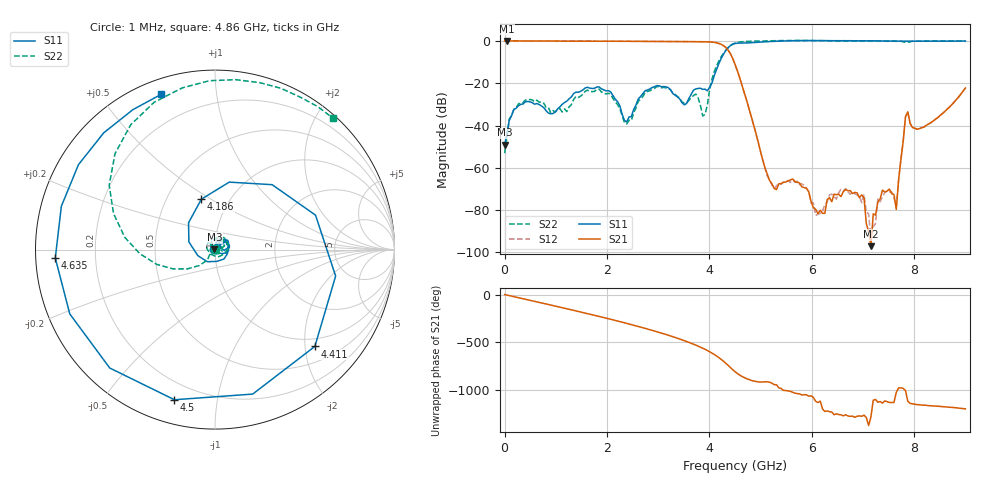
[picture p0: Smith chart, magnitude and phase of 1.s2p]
!Prosund Technologies,SP809B,SP82221046,V.03.04.C
!Date: Sunday, January 19, 2025 15:10:32
!Correction: S11(C  2-Port  )
!S21(C  2-Port  )
!S12(C  2-Port  )
!S22(C  2-Port  )
!S2P File: Measurement: :
# Hz S  dB  R 50
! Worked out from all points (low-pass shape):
!   201 points, 1 MHz to 9 GHz, reference 50 ohm
!   highest |S21| = 0.01 dB at 45.99 MHz (marker M1); lowest = -97.0 dB at 7.155 GHz (marker M2)
!   |S21| within 3 dB of the highest: start of sweep to 4.314 GHz
!   lowest |S11| = -49.0 dB at 1 MHz (marker M3), VSWR 1.01, Z = 49.7 + j0.187 ohm
!   |S11| at or under -10 dB: start of sweep to 4.199 GHz
!   |S22| runs from -53.1 to 0.2 dB; largest |S21 - S12| = 0.016
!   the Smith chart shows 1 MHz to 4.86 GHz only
!   S11 on the Smith chart (normalised r, x): 1 MHz: 0.99, +0.00; 4.186 GHz: 0.74, +0.45; 4.411 GHz: 0.82, -2.21; 4.5 GHz: 0.11, -0.76; 4.635 GHz: 0.06, -0.03; 4.86 GHz: 0.07, +0.71
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1000000  -49.04 147.7  -0.03 -0.2  -0.03 -0.1  -53.07 117.8
4.5995e7  -44.44 104.4  0.01 -5.8  0.04 -5.6  -45.85 83.3
2.7097e8  -30.66 45.1  -0.03 -32.9  0.01 -32.6  -29.76 34.0
7.65915e8  -31.55 11.4  -0.07 -92.9  -0.03 -92.6  -29.47 -38.4
1.53083e9  -23.18 42.2  -0.14 172.3  -0.11 172.8  -25.23 90.8
2.25075e9  -30.63 -40.2  -0.17 78.0  -0.15 78.6  -31.99 -8.5
3.015665e9  -21.20 32.4  -0.26 -34.2  -0.23 -33.4  -21.56 47.6
3.42062e9  -27.46 2.6  -0.31 -103.7  -0.28 -103.1  -26.95 -61.9
3.78058e9  -22.49 15.8  -0.41 -177.9  -0.39 -177.0  -26.86 129.7
3.915565e9  -22.83 -46.9  -0.43 149.0  -0.41 149.7  -34.79 174.6
4.185535e9  -10.73 105.1  -1.22 62.5  -1.20 63.4  -9.51 -165.7
4.41051e9  -2.21 -44.1  -6.04 -40.6  -6.04 -40.0  -2.25 136.2
4.5005e9  -1.25 -105.1  -11.02 -83.9  -11.01 -83.4  -1.03 112.5
4.635485e9  -1.00 -177.0  -20.85 -133.3  -20.85 -132.4  -0.41 83.0
4.86046e9  -0.77 109.1  -39.40 178.7  -39.18 178.8  -0.14 48.2
5.265415e9  -0.23 38.9  -69.71 140.2  -69.88 141.6  0.10 5.0
6.03033e9  0.16 -31.8  -78.76 7.6  -76.54 24.4  0.15 -54.4
7.155205e9  -0.00 -104.6  -97.04 163.9  -94.03 76.0  -0.02 -124.3
7.515165e9  -0.10 -122.4  -70.05 -45.2  -71.41 -36.8  -0.09 -142.0
7.65015e9  -0.11 -129.1  -79.64 60.4  -78.12 42.7  -0.11 -148.7
7.875125e9  -0.15 -139.3  -33.53 -32.7  -33.50 -31.3  -0.67 -155.9
9e9  -0.08 171.0  -22.28 -111.6  -22.29 -111.2  0.05 154.0
